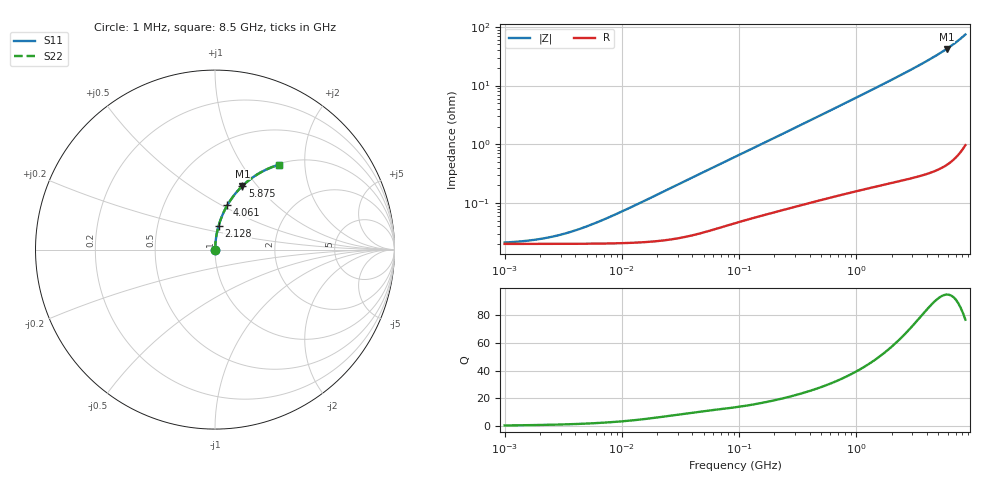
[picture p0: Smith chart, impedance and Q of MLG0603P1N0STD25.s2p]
! S-Parameter Data Generated by TDK Corporation
! Copyright(C) 2025 TDK Corporation.
! All Rights Reserved.
! TDK P/N: MLG0603P1N0STD25 (SMD / SMT Inductor (Coil))
! Property: L=1nH at 500MHz
! Size(LxWxT): 0.6x0.3x0.3mm
! Model Type: s2p (Touchstone File Format Version 1.0)
! Frequency: DC=Yes Start=1MHz Stop=8500MHz 198points Log-sweep
! Model Generated on Feb. 6, 2025
! Terms and conditions regarding TDK Simulation Models:
! 1)This simulation model is being provided solely for informational
!  purposes. Please refer to the specifications of the products in
!  terms of detailed characteristics of such products.
! 2)In no event shall TDK Corporation of any of its subsidiaries be
!  liable for any loss or damage arising, directly or indirectly,
!  from any information contained in this simulation model, including,
!  but not limited to loss or damages arising from any inaccuracies,
!  omissions or errors in connection with such information.
! 3)Any and all copyrights on this simulation model are owned by
!  TDK Corporation.  Duplication or redistribution of this simulation
!  model without prior written permission from TDK Corporation
!  is prohibited.
! 4)This simulation model is subject to any modification or change
!  without any prior notice.
! 5)Neither TDK Corporation nor any of its subsidiaries shall make any
!  warranty, express or implied, including but not limited to the
!  correctness, implied warranties of merchantability and fitness for
!  a particular purpose with respect to this simulation models.
! 6)The use of this simulation model shall be deemed to have consented
!  to the terms and conditions hereof.
! Port Assignments:
!  1 ---@@@--- 2
! Applicable Conditions:
!  Temperature = 25 degC
!  DC Bias Current = 0 A
!  Small Signal Operation
# Hz S MA R 50
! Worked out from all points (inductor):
!   197 points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, 1 MHz to 8.5 GHz, reference 50 ohm
!   read as one part in series: L = 1.09 nH near 9.169 MHz
!   highest Q = 94.9 at 5.875 GHz (marker M1), where L = 1.14 nH
!   S11 on the Smith chart (normalised r, x): 1 MHz: 1.00, +0.00; 2.128 GHz: 1.00, +0.27; 4.061 GHz: 1.01, +0.53; 5.875 GHz: 1.01, +0.84; 8.5 GHz: 1.02, +1.48
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1000000  0.0002114 18.9  0.9998 -0.0  0.9998 -0.0  0.0002114 18.9
1586648  0.0002277 28.5  0.9998 -0.0  0.9998 -0.0  0.0002277 28.5
2295435  0.0002545 38.1  0.9998 -0.0  0.9998 -0.0  0.0002545 38.1
3171038  0.0002955 47.2  0.9998 -0.0  0.9998 -0.0  0.0002955 47.2
4587603  0.0003728 57.3  0.9998 -0.0  0.9998 -0.0  0.0003728 57.3
6051655  0.0004607 63.9  0.9998 -0.0  0.9998 -0.0  0.0004607 63.9
8360083  0.000607 70.3  0.9998 -0.0  0.9998 -0.0  0.000607 70.3
2.10461e7  0.001451 81.0  0.9998 -0.1  0.9998 -0.1  0.001451 81.0
9.219544e7  0.006078 85.4  0.9995 -0.3  0.9995 -0.3  0.006078 85.4
4.229561e8  0.02664 86.3  0.9986 -1.5  0.9986 -1.5  0.02664 86.3
1.016736e9  0.06318 84.9  0.9964 -3.6  0.9964 -3.6  0.06318 84.9
1.404574e9  0.08709 83.8  0.9944 -5.0  0.9944 -5.0  0.08709 83.8
1.940355e9  0.1204 82.1  0.9906 -6.9  0.9906 -6.9  0.1204 82.1
2.128028e9  0.1321 81.4  0.989 -7.6  0.989 -7.6  0.1321 81.4
2.939772e9  0.1837 78.6  0.9804 -10.6  0.9804 -10.6  0.1837 78.6
4.061159e9  0.2574 74.4  0.9633 -14.9  0.9633 -14.9  0.2574 74.4
4.884749e9  0.3141 71.1  0.946 -18.3  0.946 -18.3  0.3141 71.1
5.87536e9  0.3854 66.7  0.9187 -22.7  0.9187 -22.7  0.3854 66.7
6.44363e9  0.428 64.1  0.8992 -25.3  0.8992 -25.3  0.428 64.1
7.066863e9  0.4761 60.9  0.8742 -28.4  0.8742 -28.4  0.4761 60.9
7.750377e9  0.5305 57.3  0.8415 -32.0  0.8415 -32.0  0.5305 57.3
8.5e9  0.5915 53.0  0.7987 -36.3  0.7987 -36.3  0.5915 53.0
